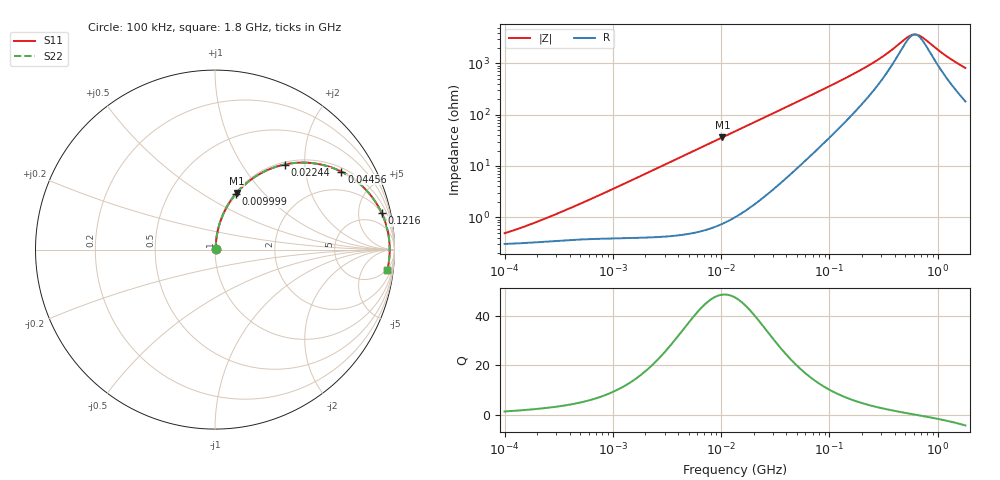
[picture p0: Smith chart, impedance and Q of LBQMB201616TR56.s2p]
! LBQMB201616TR56  S-PARAMETER MODEL  ( General Type )
! Model Generated by TAIYO YUDEN Corporation (http://www.ty-top.com)
! Version 1.0
! TAIYO YUDEN Control No. 191025NI43SB-FBB
! Copyright(c) 2019 TAIYO YUDEN CO.,LTD. All Rights Reserved.
! Product Description (link to TY-COMPAS)
! https://ds.yuden.co.jp/TYCOMPAS/or/detail?pn=LBQMB201616TR56J&u=M
! Products Name : Inductors
! Characteristics :
!  Inductance : 0.56 uH , SRF(min) : 300 MHz , DC Resistance(max) : 0.377 Ohm , Rated Current : 410 mA
!  Case Size : 2.0 x 1.6 / 0.079 x 0.063 [mm/inch] , Thickness : 1.6 / 0.063 [mm/inch]
!  (Conditions: Temperature = 25 degC , DC Bias Current/Voltage = 0A / 0V)
! External Node Assignments :
!  1  o---GGG---o  2
! GND o---------o GND
! Frequency Range : 0.1MHz  -  1800MHz  [ 402 STEP ]
# MHz S RI R 50
! Freq[MHz].  S11 Real  S11 Imag  S21 Real  S21 Imag  S12 Real  S12 Imag  S22 Real  S22 Imag
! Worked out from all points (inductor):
!   401 points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, 100 kHz to 1.8 GHz, reference 50 ohm
!   read as one part in series: L = 582 nH near 279.8 kHz
!   highest Q = 48.4 at 10.25 MHz (marker M1), where L = 560 nH
!   self-resonance near 614.8 MHz
!   S11 on the Smith chart (normalised r, x): 100 kHz: 1.01, +0.01; 9.999 MHz: 1.01, +0.70; 22.44 MHz: 1.04, +1.58; 44.56 MHz: 1.14, +3.15; 121.6 MHz: 2.07, +8.78; 1.8 GHz: 5, -16
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0.1  0.00303 0.00383  0.997 -0.00383  0.997 -0.00383  0.00303 0.00383
0.193745  0.00329 0.00725  0.9967 -0.00725  0.9967 -0.00725  0.00329 0.00725
0.516129  0.00403 0.0184  0.996 -0.0184  0.996 -0.0184  0.00403 0.0184
1.309209  0.00601 0.0458  0.994 -0.0458  0.994 -0.0458  0.00601 0.0458
2.66389  0.0127 0.0923  0.9873 -0.0923  0.9873 -0.0923  0.0127 0.0923
5.833619  0.0449 0.1951  0.9551 -0.1951  0.9551 -0.1951  0.0449 0.1951
9.999495  0.1152 0.3091  0.8848 -0.3091  0.8848 -0.3091  0.1152 0.3091
10.24746  0.1201 0.315  0.8799 -0.315  0.8799 -0.315  0.1201 0.315
13.41641  0.1875 0.3799  0.8125 -0.3799  0.8125 -0.3799  0.1875 0.3799
22.44079  0.3875 0.4741  0.6125 -0.4741  0.6125 -0.4741  0.3875 0.4741
31.62078  0.5525 0.4806  0.4475 -0.4806  0.4475 -0.4806  0.5525 0.4806
44.5561  0.7042 0.4342  0.2958 -0.4342  0.2958 -0.4342  0.7042 0.4342
69.24595  0.842 0.3319  0.158 -0.3319  0.158 -0.3319  0.842 0.3319
121.6389  0.9289 0.2029  0.0711 -0.2029  0.0711 -0.2029  0.9289 0.2029
224.4022  0.9624 0.1028  0.0376 -0.1028  0.0376 -0.1028  0.9624 0.1028
357.3983  0.9709 0.0497  0.0291 -0.0497  0.0291 -0.0497  0.9709 0.0497
528.8877  0.9733 0.0132  0.0267 -0.0132  0.0267 -0.0132  0.9733 0.0132
583.3325  0.9734 0.0046  0.0266 -0.0046  0.0266 -0.0046  0.9734 0.0046
643.382  0.9734 -0.00399  0.0266 0.00399  0.0266 0.00399  0.9734 -0.00399
745.2431  0.9732 -0.017  0.0268 0.017  0.0268 0.017  0.9732 -0.017
1246.522  0.9688 -0.0669  0.0312 0.0669  0.0312 0.0669  0.9688 -0.0669
1800  0.9604 -0.1118  0.0396 0.1118  0.0396 0.1118  0.9604 -0.1118
